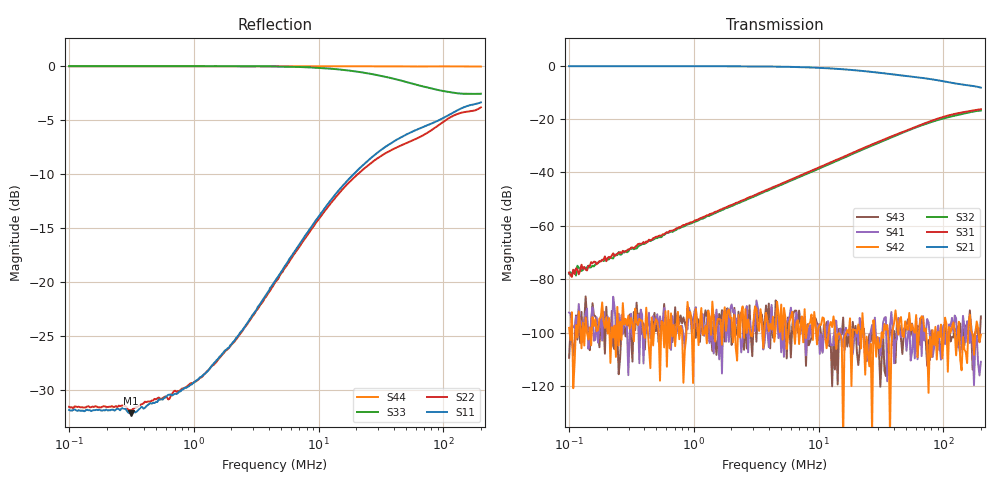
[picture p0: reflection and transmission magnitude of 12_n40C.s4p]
!Keysight Technologies,E5080A,MY55200740,A.12.60.03
!Date: Friday, October 02, 2020 16:23:22
!Correction: S11(Full 4 Port(1,2,3,4))
!S12(Full 4 Port(1,2,3,4))
!S13(Full 4 Port(1,2,3,4))
!S14(Full 4 Port(1,2,3,4))
!S21(Full 4 Port(1,2,3,4))
!S22(Full 4 Port(1,2,3,4))
!S23(Full 4 Port(1,2,3,4))
!S24(Full 4 Port(1,2,3,4))
!S31(Full 4 Port(1,2,3,4))
!S32(Full 4 Port(1,2,3,4))
!S33(Full 4 Port(1,2,3,4))
!S34(Full 4 Port(1,2,3,4))
!S41(Full 4 Port(1,2,3,4))
!S42(Full 4 Port(1,2,3,4))
!S43(Full 4 Port(1,2,3,4))
!S44(Full 4 Port(1,2,3,4))
!S4P File: Measurements: <S11,S12,S13,S14>,
!<S21,S22,S23,S24>,
!<S31,S32,S33,S34>,
!<S41,S42,S43,S44>:Log Frequency Sweep
# Hz S  dB  R 50
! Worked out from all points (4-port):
!   300 points, 100 kHz to 200 MHz, reference 50 ohm
!   strongest paths, dB at 100 kHz, 673 kHz, 4.529 MHz, 30.48 MHz, 200 MHz:
!     S21: -0.2, -0.2, -0.4, -2.7, -8.3
!     S31: -77.5, -61.8, -45.1, -28.4, -16.3
!     S32: -78.0, -62.3, -45.5, -28.8, -16.8
!     S42: -98.2, -101.4, -98.6, -105.8, -100.8
!     S41: -92.5, -93.8, -94.6, -101.9, -110.9
!     S43: -109.4, -103.5, -87.9, -107.0, -93.9
!   lowest |S11| = -32.2 dB at 313.9 kHz (marker M1), VSWR 1.05, Z = 52.5 - j0.452 ohm
!   |S11| at or under -10 dB: start of sweep to 19.11 MHz
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100000  -31.87 -0.3  -0.23 -0.1  -78.17 73.6  -92.49 -175.3
        -0.23 -0.1  -31.58 0.2  -78.86 94.3  -90.02 -30.8
        -77.47 85.6  -78.01 93.0  0.00 -0.1  -98.42 111.3
        -92.49 -54.0  -98.21 43.7  -109.43 -168.4  -0.00 -0.0
119476.3  -31.89 -1.9  -0.23 -0.2  -75.64 93.5  -96.06 36.7
          -0.23 -0.2  -31.57 -1.6  -76.27 89.4  -101.57 -11.9
          -78.15 92.4  -75.69 93.0  0.00 -0.2  -98.67 -73.3
          -89.26 -116.6  -92.07 123.0  -94.39 44.0  0.00 -0.0
313913.9  -32.18 -10.1  -0.23 -0.4  -68.67 92.1  -104.45 74.7
          -0.23 -0.4  -31.94 -9.6  -68.88 91.2  -94.46 37.9
          -68.19 92.2  -68.68 91.0  0.00 -0.4  -100.42 -5.2
          -92.92 128.8  -94.48 -51.9  -101.80 165.2  -0.00 -0.0
1442861  -27.56 -58.5  -0.24 -1.9  -55.13 89.3  -94.37 -9.0
         -0.24 -1.9  -27.70 -56.0  -55.52 89.9  -94.40 -86.6
         -55.07 89.3  -55.45 89.6  0.00 -2.0  -102.80 -96.0
         -107.80 119.1  -95.02 159.4  -93.26 47.9  0.00 -0.1
1.928983e7  -9.95 -123.9  -1.72 -15.5  -32.41 83.5  -102.17 -139.2
            -1.72 -15.5  -10.31 -114.3  -32.81 86.2  -113.57 -46.3
            -32.39 83.5  -32.80 85.9  -0.47 -24.5  -97.65 95.3
            -102.71 -131.2  -98.93 -127.4  -102.08 4.4  -0.00 -1.3
7.234702e7  -5.53 -150.4  -4.81 -19.6  -21.46 63.1  -104.36 89.0
            -4.81 -19.6  -6.26 -130.0  -21.83 70.5  -100.21 141.0
            -21.47 63.1  -21.83 70.4  -1.94 -69.9  -105.67 103.2
            -100.38 -140.0  -98.49 29.3  -103.20 47.3  -0.02 -5.0
2e8  -3.36 -162.7  -8.28 -11.7  -16.36 27.7  -99.90 -46.8
     -8.27 -11.8  -3.82 -110.4  -16.86 50.7  -95.40 146.8
     -16.34 27.7  -16.85 50.6  -2.55 -119.4  -93.21 -84.1
     -110.91 -96.5  -100.81 148.7  -93.92 -43.1  -0.03 -13.6
